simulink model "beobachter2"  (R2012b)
settings: Solver=ode45  StartTime=0.0  StopTime=10.0  RelTol=1e-3
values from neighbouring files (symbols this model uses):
  A = [0 1 0 0 0 0    [beobachter_1.m]    (also in beobachter_2.m; beobachter_22.m; kalman_1.m = my_sys.a; kalman_10.m = my_sys.a)
  B = [0 1 0 0 0 0]'    [beobachter_1.m]    (also in beobachter_2.m; beobachter_22.m; kalman_1.m = my_sys.b; kalman_10.m = my_sys.b)
  C = [0 0 0 0 1 0]    [beobachter_1.m]    (also in beobachter_2.m; beobachter_22.m; kalman_1.m = my_sys.c; kalman_10.m = my_sys.c)
  D = 0    [aktiv_tilger_1.m]    (also in aktiv_tilger_12.m; aktiv_tilger_3.m = 2000; aktiv_tilger_31.m; beobachter_1.m)
  Ke = (place(A',C',p))'    [beobachter_1.m]    (also in beobachter_2.m; beobachter_22.m)
  x0 = [30,-20,0,0,0,0]    [beobachter_1.m]    (also in beobachter_2.m = [0,0,0,0,0.3,0]; beobachter_22.m = [0.1,0,0.1,0,0.3,0]; kalman_13.m = zeros(1,3); kalman_d1.m = zeros(1,3))

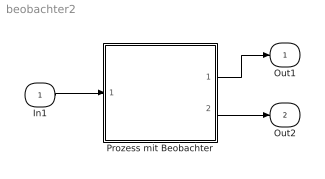
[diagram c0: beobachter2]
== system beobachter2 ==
  In1 : Inport
  Prozess mit Beobachter : Subsystem
  Out1 : Outport
  Out2 : Outport  Port=2
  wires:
  In1/1 -> Prozess mit Beobachter/1(u(t))
  Prozess mit Beobachter/1(Ausgang y(t)) -> Out1/1
  Prozess mit Beobachter/2(GeschÃ¤tzter x(t)) -> Out2/1

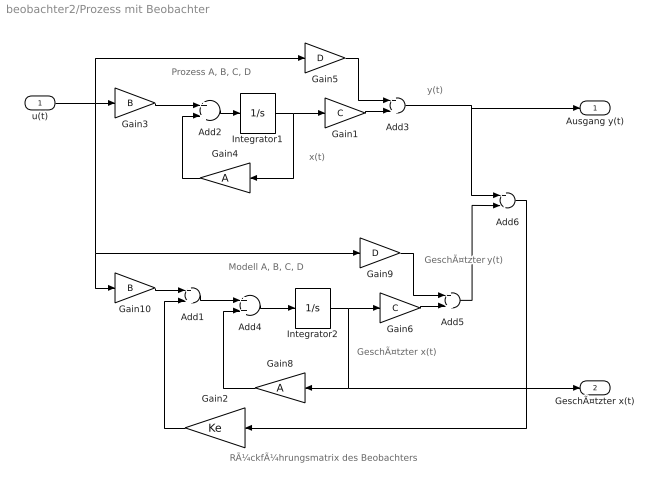
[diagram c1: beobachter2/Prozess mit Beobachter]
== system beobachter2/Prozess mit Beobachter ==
  note: GeschÃ¤tzter
  note: y(t)
  note: x(t)
  note: Prozess A, B, C, D
  note: y(t)
  note: GeschÃ¤tzter x(t)
  note: RÃ¼ckfÃ¼hrungsmatrix des Beobachters
  note: Modell A, B, C, D
  u(t) : Inport
  Add{1..5} (5 alike) : Sum
  Add6 : Sum  Inputs=+-
  Gain1 : Gain  Gain=C  Multiplication=Matrix(K*u)
  Gain10 : Gain  Gain=B  Multiplication=Matrix(K*u)
  Gain2 : Gain  Gain=Ke  Multiplication=Matrix(K*u)
  Gain3 : Gain  Gain=B  Multiplication=Matrix(K*u)
  Gain4 : Gain  Gain=A  Multiplication=Matrix(K*u)
  Gain5 : Gain  Gain=D  Multiplication=Matrix(K*u)
  Gain6 : Gain  Gain=C  Multiplication=Matrix(K*u)
  Gain8 : Gain  Gain=A  Multiplication=Matrix(K*u)
  Gain9 : Gain  Gain=D  Multiplication=Matrix(K*u)
  Integrator1 : Integrator  InitialCondition=x0
  Integrator2 : Integrator
  Ausgang y(t) : Outport
  GeschÃ¤tzter x(t) : Outport  Port=2
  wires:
  Gain6/1 -> Add5/2
  Gain8/1 -> Add4/2
  Add3/1 -> Ausgang y(t)/1, Add6/1
  Integrator1/1 -> Gain1/1, Gain4/1
  Add1/1 -> Add4/1
  Gain5/1 -> Add3/1
  Gain1/1 -> Add3/2
  Add2/1 -> Integrator1/1
  Add6/1 -> Gain2/1
  Add5/1 -> Add6/2
  Gain3/1 -> Add2/1
  Gain4/1 -> Add2/2
  Gain9/1 -> Add5/1
  Integrator2/1 -> GeschÃ¤tzter x(t)/1, Gain8/1, Gain6/1
  u(t)/1 -> Gain10/1, Gain9/1, Gain3/1, Gain5/1
  Add4/1 -> Integrator2/1
  Gain10/1 -> Add1/1
  Gain2/1 -> Add1/2
